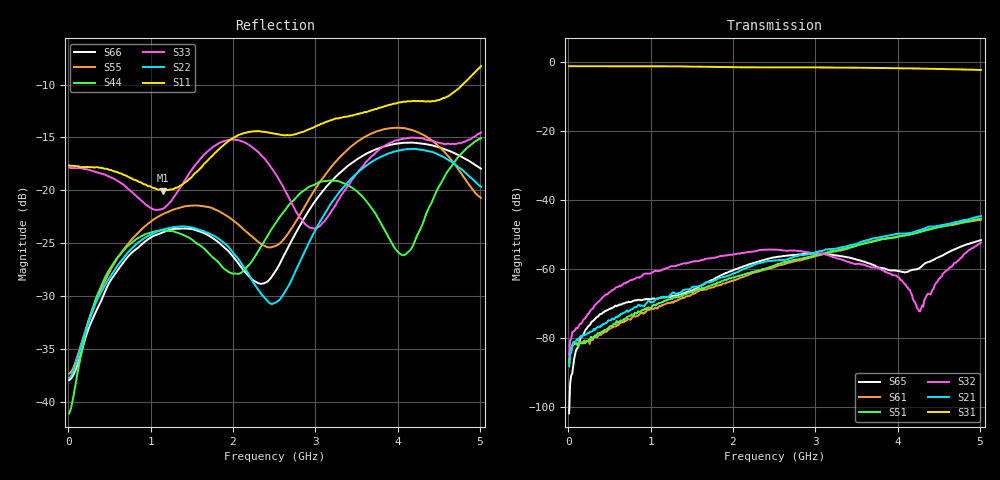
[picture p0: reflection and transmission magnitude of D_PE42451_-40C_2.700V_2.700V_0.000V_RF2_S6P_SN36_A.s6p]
! Device ID: PE42451
! Serial: 36
! Insertion: A
! Temp: -40C
! VDD: 2.700
! Control_Hi: 100.000
! Control_Lo: 0.000
! Logic State: RF2
! Port 1: RFC
! Port 2: RF1
! Port 3: RF2
! Port 4: RF3
! Port 5: RF4
! Port 6: RF5
! V1 = 0.00
! V2 = 2.70
! V3 = 0.00
! V4 = 0.00
! IDD: 1.075070e-05
#  Hz  S  RI  R  50
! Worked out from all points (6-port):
!   401 points, 10 MHz to 5.01 GHz, reference 50 ohm
!   strongest paths, dB at 10 MHz, 1.26 GHz, 2.51 GHz, 3.76 GHz, 5.01 GHz:
!     S31: -1.3, -1.4, -1.7, -1.8, -2.4
!     S21: -88.2, -67.1, -57.6, -51.0, -44.8
!     S32: -84.9, -59.3, -54.5, -59.8, -52.4
!     S51: -87.8, -68.7, -59.1, -51.8, -45.5
!     S61: -88.3, -69.6, -59.5, -51.6, -45.8
!     S65: -101.9, -67.9, -56.7, -59.6, -51.7
!   lowest |S11| = -20.0 dB at 1.147 GHz (marker M1), VSWR 1.22, Z = 57.1 - j8.02 ohm
!   |S11| at or under -10 dB: start of sweep to 4.787 GHz
